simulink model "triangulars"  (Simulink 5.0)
settings: Solver=ode45  StartTime=0.0  StopTime=10.0  RelTol=1e-3
undefined symbols (not defined in the file or in its folder): changeError, sigbuilder_block
libraries: fuzblock x8

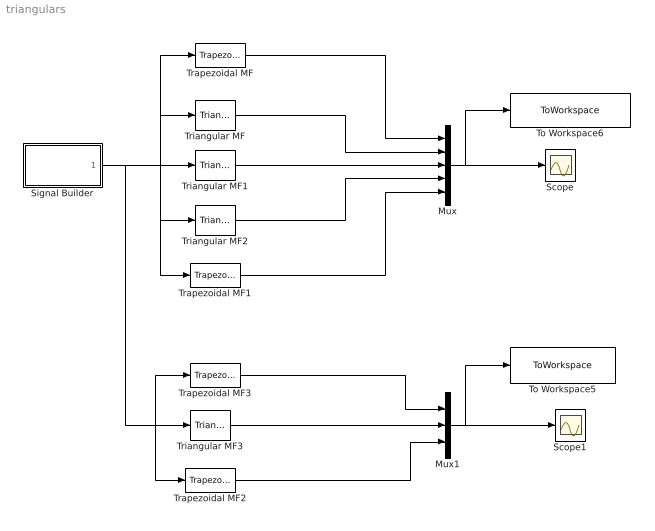
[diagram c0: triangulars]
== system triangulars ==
  Mux : Mux  Inputs=5
  Mux1 : Mux  Inputs=3
  Scope : Scope
  Scope1 : Scope
  Signal Builder : Subsystem  Tag=STV Subsys  StartFcn=sigbuilder_block('start');  StopFcn=sigbuilder_block('stop');  ClipboardFcn=sigbuilder_block('clipboard');
  To Workspace5 : ToWorkspace  VariableName=table_input_2  SampleTime=1/20  SaveFormat=Array
  To Workspace6 : ToWorkspace  VariableName=table_input_1  SampleTime=1/20  SaveFormat=Array
  Trapezoidal MF : fuzblock/Membership  Functions/Trapezoidal MF  a=changeError.input(1).mf(1).params(1)  b=changeError.input(1).mf(1).params(2)  c=changeError.input(1).mf(1).params(3)  d=changeError.input(1).mf(1).params(4)
  Trapezoidal MF1 : fuzblock/Membership  Functions/Trapezoidal MF  a=changeError.input(1).mf(5).params(1)  b=changeError.input(1).mf(5).params(2)  c=changeError.input(1).mf(5).params(3)  d=changeError.input(1).mf(5).params(4)
  Trapezoidal MF2 : fuzblock/Membership  Functions/Trapezoidal MF  a=changeError.input(2).mf(3).params(1)  b=changeError.input(2).mf(3).params(2)  c=changeError.input(2).mf(3).params(3)  d=changeError.input(2).mf(3).params(4)
  Trapezoidal MF3 : fuzblock/Membership  Functions/Trapezoidal MF  a=changeError.input(2).mf(1).params(1)  b=changeError.input(2).mf(1).params(2)  c=changeError.input(2).mf(1).params(3)  d=changeError.input(2).mf(1).params(4)
  Triangular MF : fuzblock/Membership  Functions/Triangular MF  a=changeError.input(1).mf(2).params(1)  b=changeError.input(1).mf(2).params(2)  c=changeError.input(1).mf(2).params(3)
  Triangular MF1 : fuzblock/Membership  Functions/Triangular MF  a=changeError.input(1).mf(3).params(1)  b=changeError.input(1).mf(3).params(2)  c=changeError.input(1).mf(3).params(3)
  Triangular MF2 : fuzblock/Membership  Functions/Triangular MF  a=changeError.input(1).mf(4).params(1)  b=changeError.input(1).mf(4).params(2)  c=changeError.input(1).mf(4).params(3)
  Triangular MF3 : fuzblock/Membership  Functions/Triangular MF  a=changeError.input(2).mf(2).params(1)  b=changeError.input(2).mf(2).params(2)  c=changeError.input(2).mf(2).params(3)
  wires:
  Signal Builder/1(Signal 1) -> Trapezoidal MF1/1, Triangular MF2/1, Triangular MF1/1, Triangular MF/1, Trapezoidal MF/1, Trapezoidal MF2/1, Trapezoidal MF3/1, Triangular MF3/1
  Trapezoidal MF/1 -> Mux/1
  Triangular MF/1 -> Mux/2
  Triangular MF1/1 -> Mux/3
  Mux/1 -> Scope/1, To Workspace6/1
  Trapezoidal MF1/1 -> Mux/5
  Mux1/1 -> Scope1/1, To Workspace5/1
  Trapezoidal MF3/1 -> Mux1/1
  Triangular MF3/1 -> Mux1/2
  Trapezoidal MF2/1 -> Mux1/3
  Triangular MF2/1 -> Mux/4

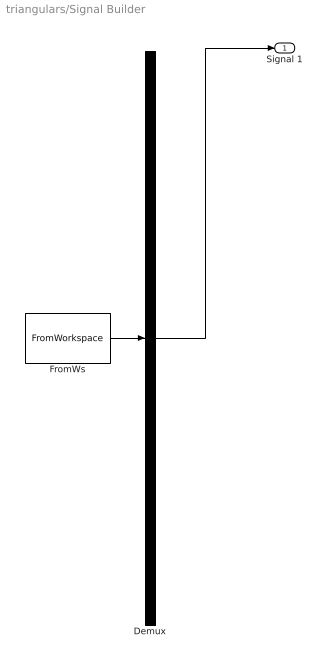
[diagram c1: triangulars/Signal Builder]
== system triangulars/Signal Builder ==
  Demux : Demux  Tag=STV Demux  Outputs=1
  FromWs : FromWorkspace  Tag=STV FromWs  VariableName=tuvar  SampleTime=0  SigBuilderData=DataTag0
  Signal 1 : Outport  Tag=STV Outport
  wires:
  Demux/1 -> Signal 1/1
  FromWs/1 -> Demux/1
